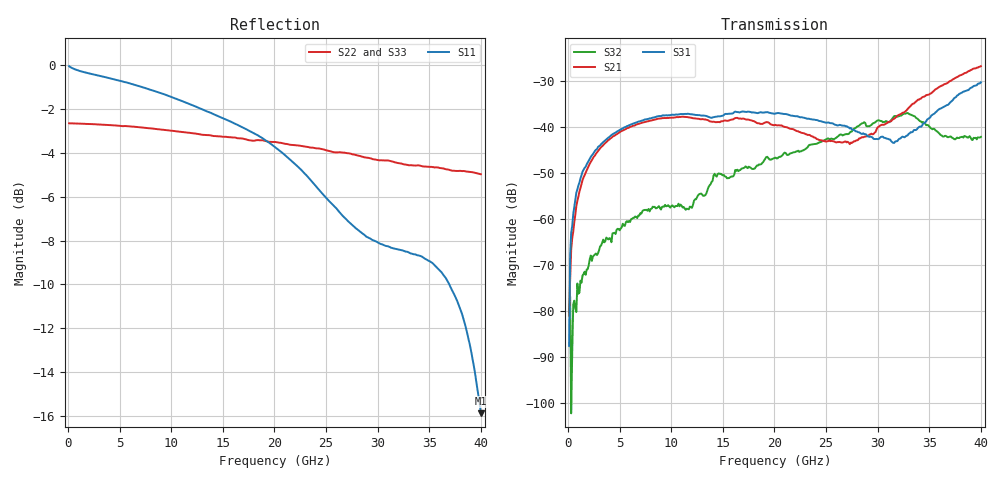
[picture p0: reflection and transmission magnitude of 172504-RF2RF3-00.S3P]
!  3-Port S-parameters saved by WinCal
! VAR MeasName=S-Parameters (CALIBRATED_DATA) read from VNA (N5245A)
! VAR MeasDate=2017-3-15 11:03:34
! VAR NAME=172504-RF2RF3-00
! VAR FILENAME=172504-RF2RF3-00.S3P
! VAR DATE=2017-3-15 11:03:34
! VAR PHYS_PORTS=1,2,3
# Hz S DB R 50
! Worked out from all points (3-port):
!   400 points, 100 MHz to 40 GHz, reference 50 ohm
!   strongest paths, dB at 100 MHz, 10.1 GHz, 20.1 GHz, 30.1 GHz, 40 GHz:
!     S31: -87.6, -37.4, -37.1, -42.7, -30.4
!     S21: -81.1, -38.1, -39.6, -40.0, -26.9
!     S32: -80.3, -57.1, -46.7, -38.6, -42.2
!   lowest |S11| = -15.9 dB at 40 GHz (marker M1), VSWR 1.38, Z = 37.7 - j7 ohm
!   |S11| at or under -10 dB: 36.94 GHz to end of sweep
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1e8  -0.06 -1.8  -85.53 102.9  -75.49 140.0
     -81.08 77.0  -2.66 179.8  -88.26 -127.2
     -87.65 58.5  -80.30 -66.1  -2.64 179.8
3e8  -0.12 -4.9  -69.60 110.4  -63.08 111.3
     -66.78 97.8  -2.66 179.3  -84.50 -159.5
     -63.08 110.0  -102.30 -161.0  -2.64 179.4
8e8  -0.23 -12.1  -57.83 96.0  -54.77 88.3
     -57.27 97.5  -2.67 178.2  -76.49 98.5
     -54.36 88.2  -80.29 113.7  -2.65 178.3
2.9e9  -0.49 -40.5  -45.34 67.0  -44.60 59.4
       -45.30 66.9  -2.71 173.8  -66.56 82.9
       -44.43 59.3  -67.55 92.7  -2.69 174.0
6.8e9  -0.96 -87.5  -39.51 28.2  -39.03 25.0
       -39.44 27.9  -2.83 165.7  -59.57 72.6
       -38.93 24.9  -59.33 72.5  -2.80 166.2
1.18e10  -1.79 -136.1  -38.01 -13.8  -37.26 -14.6
         -38.01 -13.7  -3.10 155.5  -57.47 69.3
         -37.27 -14.7  -57.39 69.5  -3.05 156.3
2.01e10  -3.76 149.8  -39.69 -57.1  -37.11 -61.8
         -39.63 -56.3  -3.51 137.7  -46.77 40.8
         -37.14 -61.5  -46.74 40.1  -3.48 138.5
2.97e10  -8.01 13.7  -41.17 -42.4  -42.44 -101.4
         -41.34 -42.5  -4.31 113.1  -39.16 -24.1
         -42.71 -99.7  -39.16 -24.0  -4.32 113.7
3.53e10  -9.02 -68.6  -32.19 -67.7  -37.11 -80.1
         -32.55 -65.6  -4.66 97.3  -40.43 -108.4
         -37.44 -77.6  -40.59 -108.4  -4.92 97.8
4e10  -15.87 -145.8  -26.63 -117.0  -30.25 -116.9
      -26.87 -114.4  -4.98 81.4  -42.51 -137.7
      -30.39 -112.5  -42.23 -136.3  -5.26 82.6
